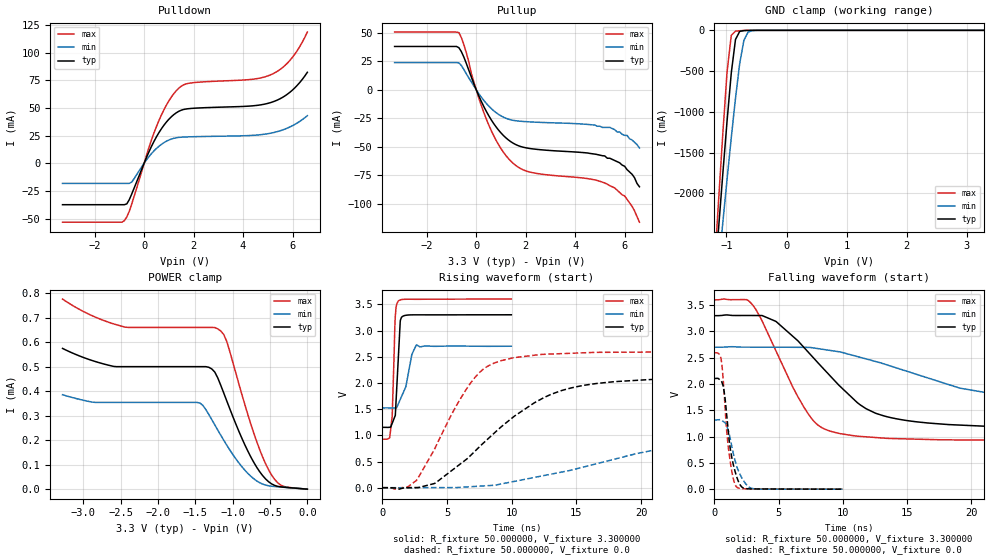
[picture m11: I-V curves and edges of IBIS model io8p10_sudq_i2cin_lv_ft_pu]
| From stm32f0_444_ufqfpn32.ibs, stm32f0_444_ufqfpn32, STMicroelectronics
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|   Model io8p10_sudq_i2cin_lv_ft_pu
[Model]  io8p10_sudq_i2cin_lv_ft_pu
Model_type I/O
Polarity   Non-Inverting
Enable   Active-Low
Vinl =   0.990000V
Vinh =   2.310000V
Vmeas =  1.650000V
Cref =   50.000000pF
Rref =   100.000000M
Vref =   0.0V
C_comp   2.070000pF   1.996000pF   2.160200pF
[Temperature Range]   25.000000   0.125000k   -40.000000
[Pullup Reference]   3.300000V   2.700000V   3.600000V
[Pulldown Reference]   0.0V   0.0V   0.0V
[POWER Clamp Reference]   3.300000V   2.700000V   3.600000V
[GND Clamp Reference]   0.0V   0.0V   0.0V
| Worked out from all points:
|   slope of the pulldown table from 0 to 0.495 V, typ, clamps not added: 20.9 ohm
|   slope of the pullup table from 0 to 0.495 V, typ, clamps not added: 22.2 ohm
|   GND clamp passes 1 mA (typ) near -0.64 V on its own axis
|   rising waveform, R_fixture 50.000000, V_fixture 3.300000: 20-80 % time 274ps typ, 706ps min, 191ps max; typ from 1.15 V to 3.3 V
|   rising waveform, R_fixture 50.000000, V_fixture 0.0: 20-80 % time 6.36ns typ, 15.1ns min, 3.52ns max; typ from 0.001 V to 2.1 V
|   falling waveform, R_fixture 50.000000, V_fixture 3.300000: 20-80 % time 5.22ns typ, 11ns min, 3.26ns max; typ from 3.3 V to 1.15 V
|   falling waveform, R_fixture 50.000000, V_fixture 0.0: 20-80 % time 671ps typ, 883ps min, 550ps max; typ from 2.1 V to 0.001 V
[Pulldown]
|Voltage   I(typ)   I(min)   I(max)
-3.3V     -37.45mA   -18.2mA    -53.24mA
-800mV    -37.45mA   -18.2mA    -51.9mA
-700mV    -36.7mA    -18.2mA    -48.48mA
-500mV    -27.71mA   -17.01mA   -36.66mA
500mV     23.91mA    13.38mA    33.24mA
900mV     37.17mA    19.88mA    52.48mA
1.3V      45.55mA    23.01mA    65.5mA
1.8V      49.29mA    23.83mA    72.18mA
4.4V      51.88mA    25.21mA    75.91mA
5.2V      55.41mA    27.53mA    80.72mA
5.9V      64.2mA     32.82mA    93.01mA
6.6V      82.13mA    42.97mA    118.5mA
[Pullup]
|Voltage   I(typ)   I(min)   I(max)
-3.3V     37.85mA    23.75mA    50.43mA
-700mV    36.77mA    23.48mA    49.96mA
-500mV    28.57mA    17.67mA    39.46mA
0V        90fA       16pA       0A
400mV     -18.61mA   -11.78mA   -25.23mA
900mV     -35.28mA   -21.54mA   -48mA
1.4V      -45.54mA   -26.4mA    -62.54mA
2.2V      -51.57mA   -28.22mA   -72.25mA
5.3V      -60mA      -33mA      -82.7mA
6V        -67mA      -40mA      -93mA
6.3V      -74mA      -44mA      -102mA
6.6V      -85mA      -51mA      -116mA
[GND_clamp]
|Voltage   I(typ)   I(min)   I(max)
-3.3V     -9.366A    -9.678A    -9.859A
-1.2V     -3.091A    -3.431A    -2.911A
-1.13V    -2.415A    -2.888A    -2.072A
-1.06V    -1.751A    -2.352A    -1.259A
-990mV    -1.112A    -1.826A    -509.3mA
-920mV    -522.9mA   -1.315A    -61.61mA
-850mV    -112.5mA   -833.8mA   -10.22mA
-780mV    -13.59mA   -408.1mA   -5.256mA
-710mV    -3.081mA   -122.1mA   -2.635mA
-640mV    -945.2uA   -21.36mA   -905.7uA
-570mV    -199.6uA   -4.142mA   -156.8uA
3.28V     0A         0A         0A
[POWER_clamp]
|Voltage   I(typ)   I(min)   I(max)
-3.28V    574uA      385.1uA    775.2uA
-2.88V    524.3uA    354.9uA    706.9uA
-2.44V    499.5uA    353.8uA    660.7uA
-1.44V    499.5uA    351.5uA    659.5uA
-1.28V    490.2uA    283.5uA    659.5uA
-1.16V    423.6uA    220uA      645uA
-1.08V    360.3uA    179.6uA    602.6uA
-800mV    157uA      65.19uA    307.1uA
-640mV    71.83uA    26.55uA    162.4uA
-520mV    30.52uA    13.8uA     79.51uA
-360mV    9.625uA    8.656uA    17.31uA
0V        0A         0A         0A
[Ramp]
| variable   typ   min   max
dV/dt_r  1.26192/6.35669n   0.77962/15.04639n   1.55439/3.51497n
dV/dt_f  1.28868/5.21287n   0.69810/11.04156n   1.60393/3.25804n
R_load = 50.000000
[Rising Waveform]
R_fixture= 50.000000
V_fixture= 3.300000
V_fixture_min= 2.700000
V_fixture_max= 3.600000
|time   V(typ)   V(min)   V(max)
0s        1.152V     1.524V     926.8mV
580.6ps   1.154V     1.523V     978.2mV
760.8ps   1.23V      1.522V     1.372V
1.001ns   1.381V     1.523V     3.268V
1.221ns   2.415V     1.594V     3.56V
1.401ns   3.204V     1.696V     3.585V
1.822ns   3.291V     1.934V     3.596V
2.282ns   3.298V     2.544V     3.596V
2.643ns   3.299V     2.727V     3.596V
9.97ns    3.3V       2.7V       3.6V
[Rising Waveform]
R_fixture= 50.000000
V_fixture= 0.0
V_fixture_min= 0.0
V_fixture_max= 0.0
|time   V(typ)   V(min)   V(max)
0s        1.067mV    1.203mV    1.031mV
2.603ns   3.92mV     -2.364mV   133.8mV
4.104ns   91.02mV    2.842mV    772.7mV
7.007ns   661mV      22.6mV     2.059V
8.208ns   942.9mV    40.85mV    2.327V
10.11ns   1.347V     116.9mV    2.479V
13.81ns   1.851V     296.9mV    2.558V
18.02ns   2.026V     549.6mV    2.585V
30.23ns   2.099V     1.115V     2.592V
49.85ns   2.105V     1.317V     2.592V
[Falling Waveform]
R_fixture= 50.000000
V_fixture= 3.300000
V_fixture_min= 2.700000
V_fixture_max= 3.600000
|time   V(typ)   V(min)   V(max)
0s        3.3V       2.7V       3.6V
2.903ns   3.303V     2.701V     3.525V
4.805ns   3.188V     2.701V     2.623V
7.307ns   2.606V     2.697V     1.433V
8.308ns   2.339V     2.664V     1.179V
9.81ns    1.951V     2.61V      1.056V
12.51ns   1.45V      2.431V     983.6mV
16.62ns   1.259V     2.116V     946.1mV
23.92ns   1.183V     1.722V     930.3mV
49.85ns   1.152V     1.524V     926.8mV
[Falling Waveform]
R_fixture= 50.000000
V_fixture= 0.0
V_fixture_min= 0.0
V_fixture_max= 0.0
|time   V(typ)   V(min)   V(max)
0s        2.105V     1.317V     2.592V
520.5ps   2.063V     1.316V     2.471V
760.8ps   1.848V     1.275V     1.818V
940.9ps   1.447V     1.209V     1.148V
1.081ns   1.094V     1.119V     798.1mV
1.421ns   522.4mV    735.6mV    254mV
1.722ns   246.5mV    451.4mV    43.22mV
2.142ns   39.86mV    211.7mV    9.815mV
2.963ns   5.793mV    12.67mV    6.573mV
9.97ns    1.067mV    1.203mV    1.031mV
